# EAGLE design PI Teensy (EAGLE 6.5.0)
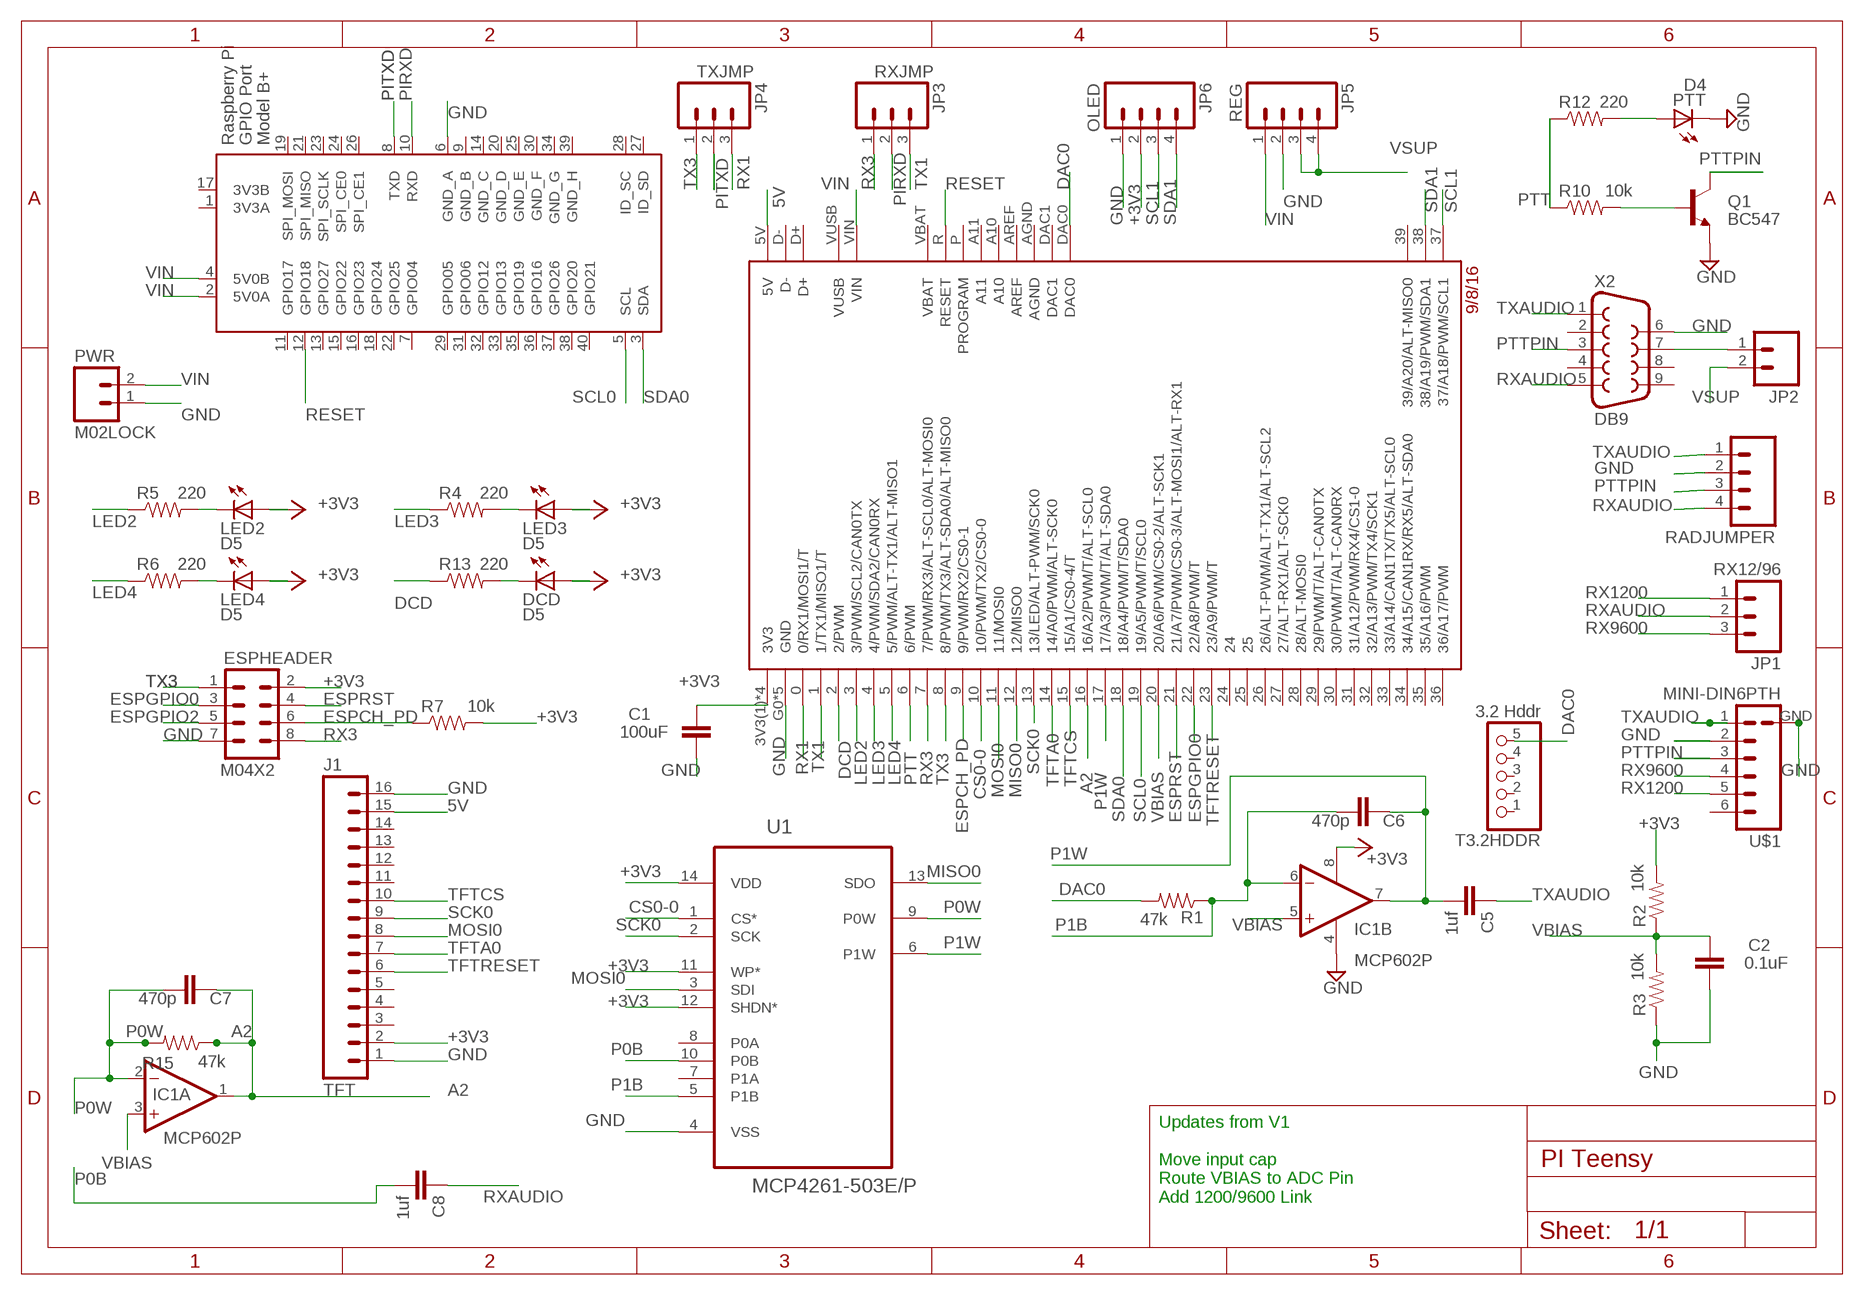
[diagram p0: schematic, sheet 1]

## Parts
C1  100uF  CAP_  [AXIAL-5MM]
C2  0.1uF  CAP_  [AXIAL-5MM]
C5  1uf  CAP_  [AXIAL-5MM]
C6  470p  CAP_  [AXIAL-5MM]
C7  470p  CAP_  [AXIAL-5MM]
C8  1uf  CAP_  [AXIAL-5MM]
DCD  D5  LED3MM  [LED3MM]
ESPHEADER  M04X2  [2X4]
IC1  MCP602P  [DIL08]
J1  TFT  M16LOCK  [1X16_LOCK]
JP1  RX12/96  M03LOCK  [1X03_LOCK]
JP2  M02LOCK  [1X02_LOCK]
JP3  RXJMP  M03LOCK  [1X03_LOCK]
JP4  TXJMP  M03LOCK  [1X03_LOCK]
JP5  REG  M04LOCK_LONGPADS  [1X04_LOCK_LONGPADS]
JP6  OLED  M04LOCK_LONGPADS  [1X04_LOCK_LONGPADS]
LED2  D5  LED3MM  [LED3MM]
LED3  D5  LED3MM  [LED3MM]
LED4  D5  LED3MM  [LED3MM]
PTT  D4  LED3MM  [LED3MM]
PWR  M02LOCK  [1X02_LOCK]
Q1  BC547  TRANSISTOR_NPNBC547  [TO-92-AMMO]
R1  47k  RESISTORAXIAL-0.3  [AXIAL-0.3]
R2  10k  RESISTOREZ  [AXIAL-0.3EZ]
R3  10k  RESISTORAXIAL-0.3  [AXIAL-0.3]
R4  220  RESISTORPTH-1/6W  [1/6W-RES]
R5  220  RESISTORPTH-1/6W  [1/6W-RES]
R6  220  RESISTORPTH-1/6W  [1/6W-RES]
R7  10k  RESISTORPTH-1/6W  [1/6W-RES]
R10  10k  RESISTORAXIAL-0.3  [AXIAL-0.3]
R12  220  RESISTORPTH-1/6W  [1/6W-RES]
R13  220  RESISTORPTH-1/6W  [1/6W-RES]
R15  47k  RESISTORAXIAL-0.3  [AXIAL-0.3]
RADJUMPER  M04LOCK  [1X04_LOCK]
T3.2HDDR  3.2 Hddr  PINHD-1X5  [1X05]
U1  MCP4261-503E/P  [DIP254P762X533-14]
U$1  MINI-DIN6PTH  [MINI-DIN6]
U$2  TEENSY3_6--ALLPINS  [T36]
X1  RASPI_BOARD_B+#_FP  [RASPI_BOARD_B+_FULL_PAD]
X2  DB9  DB9FEMALE  [DB9]

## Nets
5V [power]: J1.15 U$2.5V
+3V3 [3v3]: C1.P$1 DCD.A ESPHEADER.2 IC1.8(P:V+) J1.2 JP6.2 LED2.A LED3.A LED4.A R2.P$2 R7.2 U1.11(WP*) U1.12(SHDN*) U1.14(VDD) U$2.3V3(1)(3V3) U$2.3V3(2)(3V3) U$2.3V3(3)(3V3) U$2.3V3(4)(3V3)
A2: C7.P$1 IC1.1(A:OUT) R15.P$1 U$2.16(16/A2/PWM/T/ALT-SCL0)
CS0-0: U1.1(CS*) U$2.10(10/PWM/TX2/CS0-0)
DAC0: R1.P$2 T3.2HDDR.5 U$2.DAC0
DCD: R13.1 U$2.2(2/PWM)
ESPCH_PD: ESPHEADER.6 R7.1 U$2.9(9/PWM/RX2/CS0-1)
ESPGPIO0: ESPHEADER.3 U$2.22(22/A8/PWM/T)
ESPGPIO2: ESPHEADER.5
ESPRST: ESPHEADER.4 U$2.21(21/A7/PWM/CS0-3/ALT-MOSI1/ALT-RX1)
GND: C1.P$2 C2.P$2 ESPHEADER.7 IC1.4(P:V-) J1.1 J1.16 JP5.2 JP6.1 PTT.K(C) PWR.1 Q1.3(E) R3.P$1 RADJUMPER.2 U1.4(VSS) U$1.2 U$1.GND U$2.G0(GND) U$2.G1(GND) U$2.G2(GND) U$2.G4(GND) U$2.G5(GND) X1.6(GND_A) X2.6
LED2: R5.1 U$2.3(3/PWM/SCL2/CAN0TX)
LED3: R4.1 U$2.4(4/PWM/SDA2/CAN0RX)
LED4: R6.1 U$2.5(5/PWM/ALT-TX1/ALT-MISO1)
MISO0: U1.13(SDO) U$2.12(12/MISO0)
MOSI0: J1.8 U1.3(SDI) U$2.11(11/MOSI0)
N$1: PTT.A R12.2
N$2: Q1.2(B) R10.P$2
N$3: LED4.K(C) R6.2
N$4 [power]: JP2.1 X2.7
N$5: LED3.K(C) R4.2
N$6: LED2.K(C) R5.2
N$13: DCD.K(C) R13.2
P0B: C8.P$2 U1.10(P0B)
P0W: C7.P$2 IC1.2(A:-IN) R15.P$2 U1.9(P0W)
P1B: C6.P$2 IC1.6(B:-IN) R1.P$1 U1.5(P1B)
P1W: C5.P$2 C6.P$1 IC1.7(B:OUT) U1.6(P1W) U$2.17(17/A3/PWM/T/ALT-SDA0)
PIRXD: JP3.2 X1.10(RXD)
PITXD: JP4.2 X1.8(TXD)
PTT: R10.P$1 R12.1 U$2.6(6/PWM)
PTTPIN: Q1.1(C) RADJUMPER.3 U$1.3 X2.3
RESET: U$2.R(RESET) X1.12(GPIO18)
RX1: JP4.3 U$2.0(0/RX1/MOSI1/T)
RX3: ESPHEADER.8 JP3.1 U$2.7(7/PWM/RX3/ALT-SCL0/ALT-MOSI0)
RX1200: JP1.1 U$1.5
RX9600: JP1.3 U$1.4
RXAUDIO: C8.P$1 JP1.2 RADJUMPER.4 X2.5
SCK0: J1.9 U1.2(SCK) U$2.13(13/LED/ALT-PWM/SCK0)
SCL0: U$2.19(19/A5/PWM/T/SCL0) X1.5(SCL)
SCL1: JP6.3 U$2.37(37/A18/PWM/SCL1)
SDA0: U$2.18(18/A4/PWM/T/SDA0) X1.3(SDA)
SDA1: JP6.4 U$2.38(38/A19/PWM/SDA1)
TFTA0: J1.7 U$2.14(14/A0/PWM/ALT-SCK0)
TFTCS: J1.10 U$2.15(15/A1/CS0-4/T)
TFTRESET: J1.6 U$2.23(23/A9/PWM/T)
TX1: JP3.3 U$2.1(1/TX1/MISO1/T)
TX3: ESPHEADER.1 JP4.1 U$2.8(8/PWM/TX3/ALT-SDA0/ALT-MISO0)
TXAUDIO: C5.P$1 RADJUMPER.1 U$1.1 X2.1
VBIAS: C2.P$1 IC1.3(A:+IN) IC1.5(B:+IN) R2.P$1 R3.P$2 U$2.20(20/A6/PWM/CS0-2/ALT-SCK1)
VIN [power]: JP5.1 PWR.2 U$2.VIN X1.2(5V0A) X1.4(5V0B)
VSUP [power]: JP2.2 JP5.3 JP5.4
Unconnected: J1.3 J1.4 J1.5 J1.11 J1.12 J1.13 J1.14 T3.2HDDR.1 T3.2HDDR.2 T3.2HDDR.3 T3.2HDDR.4 U1.7(P1A) U1.8(P0A) U$1.6 U$2.24 U$2.25 U$2.26(26/ALT-PWM/ALT-TX1/ALT-SCL2) U$2.27(27/ALT-RX1/ALT-SCK0) U$2.28(28/ALT-MOSI0) U$2.29(29/PWM/T/ALT-CAN0TX) U$2.30(30/PWM/T/ALT-CAN0RX) U$2.31(31/A12/PWM/RX4/CS1-0) U$2.32(32/A13/PWM/TX4/SCK1) U$2.33(33/A14/CAN1TX/TX5/ALT-SCL0) U$2.34(34/A15/CAN1RX/RX5/ALT-SDA0) U$2.35(35/A16/PWM) U$2.36(36/A17/PWM) U$2.39(39/A20/ALT-MISO0) U$2.A10 U$2.A11 U$2.AGND U$2.AREF U$2.D+ U$2.D- U$2.DAC1 U$2.P(PROGRAM) U$2.VBAT U$2.VUSB X1.7(GPIO04) X1.11(GPIO17) X1.13(GPIO27) X1.15(GPIO22) X1.16(GPIO23) X1.18(GPIO24) X1.19(SPI_MOSI) X1.21(SPI_MISO) X1.22(GPIO25) X1.23(SPI_SCLK) X1.24(SPI_CE0) X1.26(SPI_CE1) X1.27(ID_SD) X1.28(ID_SC) X1.29(GPIO05) X1.31(GPIO06) X1.32(GPIO12) X1.33(GPIO13) X1.35(GPIO19) X1.36(GPIO16) X1.37(GPIO26) X1.38(GPIO20) X1.40(GPIO21) X2.2 X2.4 X2.8 X2.9

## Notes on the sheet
- Updates from V1
  
  Move input cap
  Route VBIAS to ADC Pin
  Add 1200/9600 Link

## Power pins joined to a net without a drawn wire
3V3A: X1.1(3V3A)
3V3B: X1.17(3V3B)
GND_B: X1.9(GND_B)
GND_C: X1.14(GND_C)
GND_D: X1.20(GND_D)
GND_E: X1.25(GND_E)
GND_F: X1.30(GND_F)
GND_G: X1.34(GND_G)
GND_H: X1.39(GND_H)

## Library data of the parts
C1 C2 C5-C8 = SparkFun-Passives:CAP: Capacitor
DCD LED2-LED4 PTT = led:LED: LED
ESPHEADER = SparkFun-Connectors:M04X2: .1" header, two rows of four.
IC1 = linear:MCP602: Single Op Amp 2.7V to 6.0V Single Supply CMOS Source: http://ww1.microchip.com/downloads/en/DeviceDoc/21314g.pdf
J1 = SparkFun-Connectors:M16: 1x16 .1" header
JP1 JP3 JP4 = SparkFun-Connectors:M03: Header 3 Standard 3-pin 0.1" header. Use with straight break away headers (SKU : PRT-00116), right angle break away headers (PRT-00553), swiss pins (PRT-00743), machine pins (PRT-00117), and female headers (PRT-00115). Molex polarized connector foot print use with SKU : PRT-08232 with associated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
JP2 PWR = SparkFun-Connectors:M02: Standard 2-pin 0.1" header. Use with
JP5 JP6 RADJUMPER = SparkFun-Connectors:M04: Header 4 Standard 4-pin 0.1" header. Use with straight break away headers (SKU : PRT-00116), right angle break away headers (PRT-00553), swiss pins (PRT-00743), machine pins (PRT-00117), and female headers (PRT-00115). Molex polarized connector foot print use with SKU : PRT-08231 with associated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
Q1 = SparkFun-DiscreteSemi:TRANSISTOR_NPN: Generic NPN BJT MMBT2222A - TRANS-08049 (SOT-23, 1A 40V) MPSA42 - TRANS-09116 (SOT-23, 500mA 300V) MMBT5088LT1G - TRANS-11160 (SOT-23, 50 mA 30V) BC547 - COM-08928 (TO-92 45V 100mA) (1.Collector 2.Base 3.Emitter) 2N3904 - COM-00521 (TO-92 40V 200mA) (1.Emitter 2.Base 3.Collector) P2N2222A -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
R1-R7 R10 R12 R13 R15 = SparkFun-Resistors:RESISTOR: Resistor
T3.2HDDR = pinhead:PINHD-1X5: PIN HEADER
U1 = MCP4261:MCP4261-503E/P: IC DGTL POT 50K 2CH ,DIP-14; MPN: MCP4261-503E/P; OC_FARNELL: 1840731; OC_NEWARK: 27M0192; PACKAGE: DIP-14; SUPPLIER: Microchip
U$1 = SparkFun-Connectors:MINI-DIN6: mini DIN 6 Connector Commonly found on the back of a computer for PS2 keyboard and mice. Schematic and footprint are proven. Spark Fun Electronics SKU : PRT-08509
U$2 = Teensy_3_6:TEENSY3_6--ALLPINS
X1 = raspberrypi_bastelstube_v13:RASPI_BOARD_B+#: Raspberry Pi GPIO connector with markings for the outer dimensions of the Raspberry Pi board model B+ with different sets of drill holes or mounting pads All pins connected
X2 = SparkFun-Connectors:DB9: DB9 Connector Standard DB9 (D-Sub 9) serial connector. Can be used for CAN bus as well as RS485 and RS232. Footprint production proven. Spark Fun Electronics SKU : PRT-00429

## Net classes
1 power: width 0.406 mm
2 3v3: width 0.305 mm

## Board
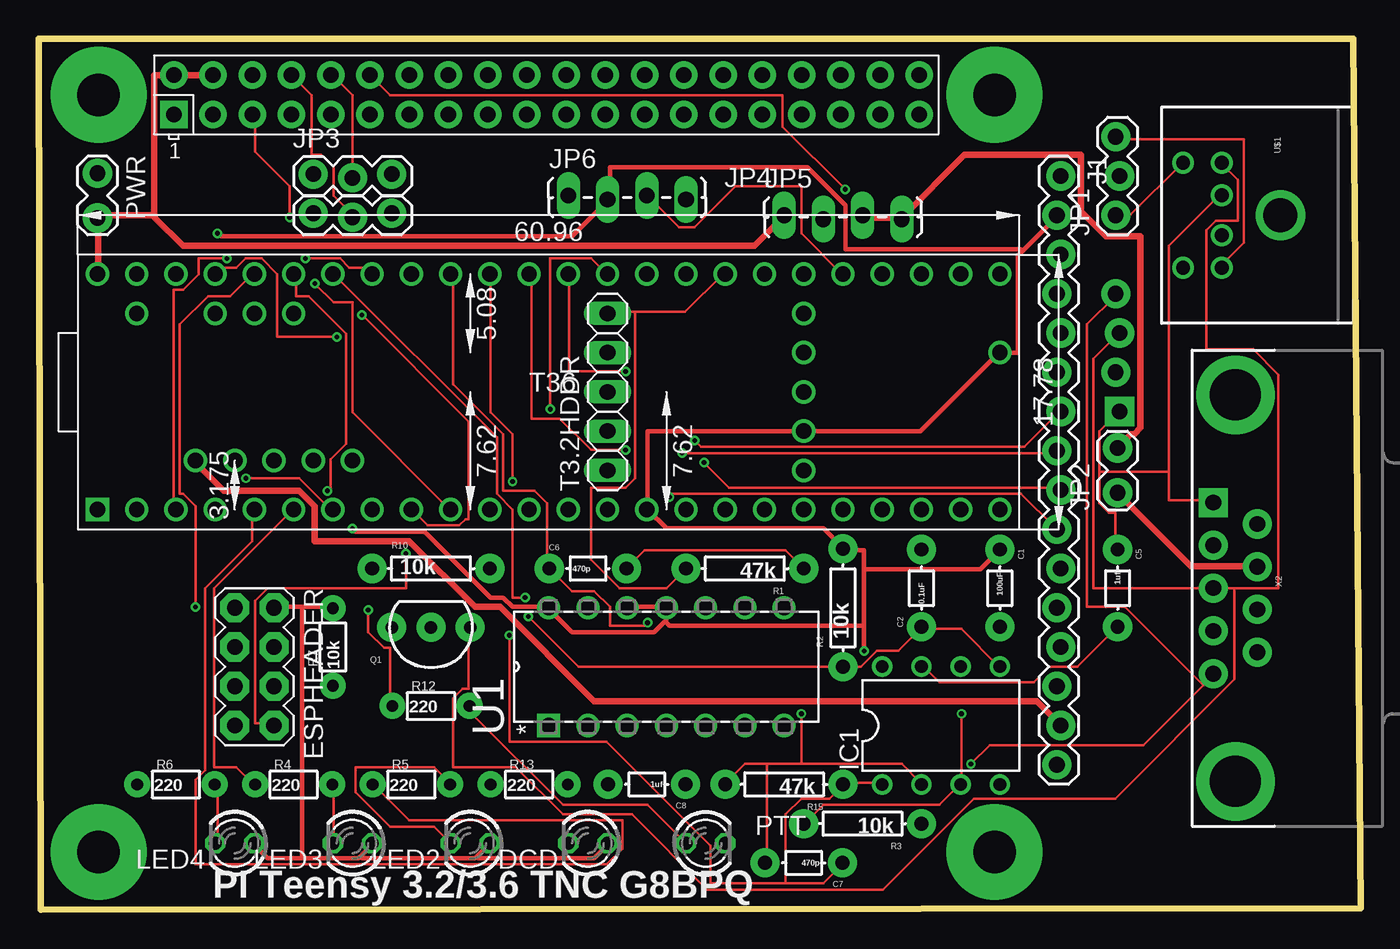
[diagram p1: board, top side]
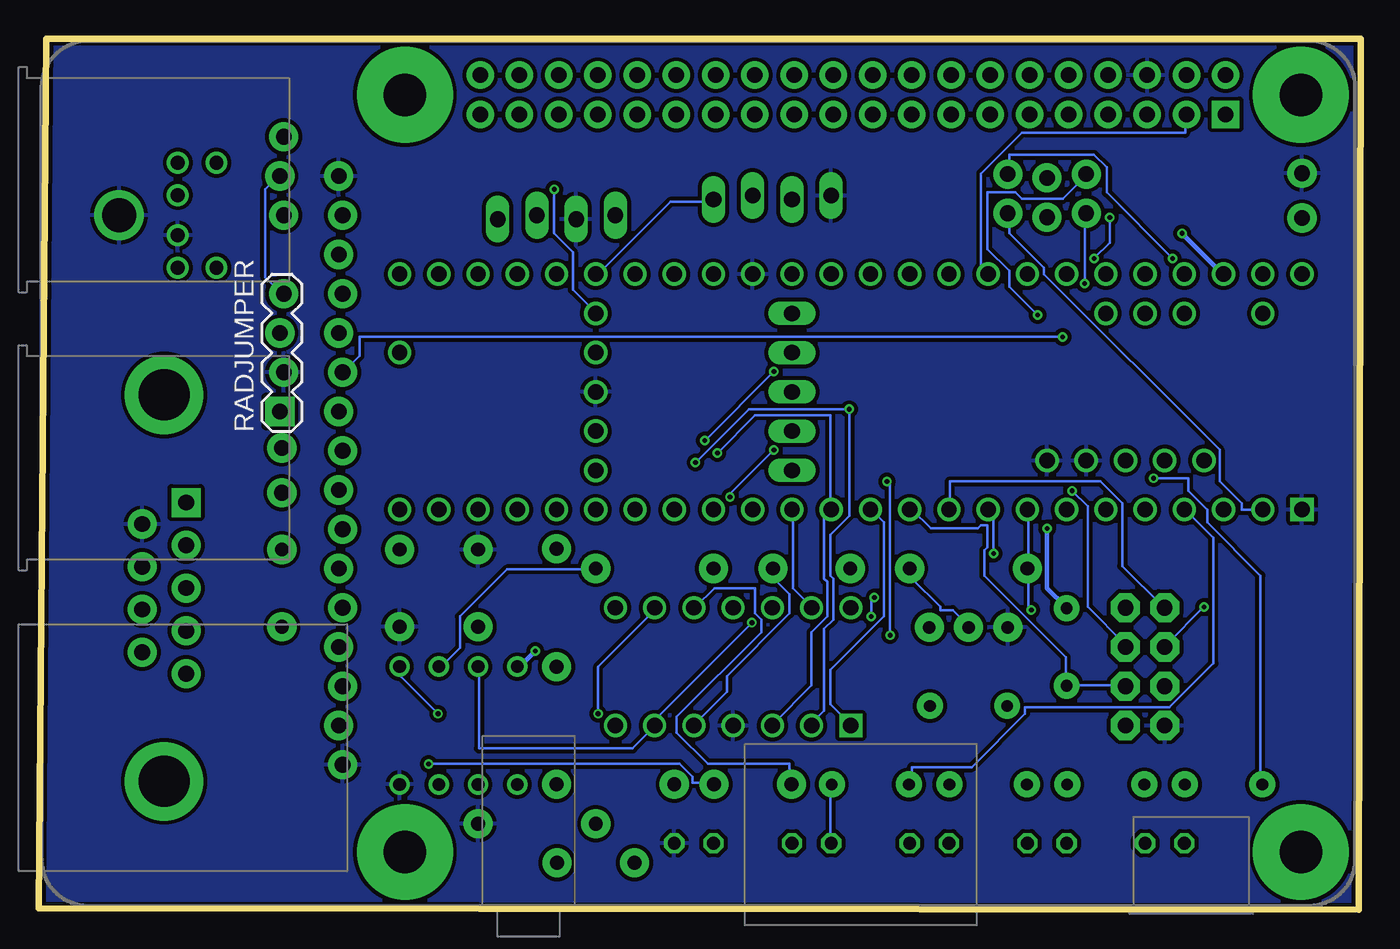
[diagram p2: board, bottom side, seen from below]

Size 85.6 x 56.39 mm. Coordinates in mm from the lower left corner, seen from the top.
Outline: 0,56.39 85.09,56.39 85.6,0.13 0.13,0 0,56.39
Copper layers (1*16): Top 0.035mm / dielectric 1.5mm / Bottom 0.035mm
Design rules "SeeedStudio_2layer_DRU_no_angle_20140221": minimum track width 6mil, minimum drill 12mil, track to track 6mil, track to pad 6mil, pad to pad 6mil, via to via 6mil, smd to smd 0mil, copper to edge 10mil, drill to drill 10mil, minimum pad ring 10mil, minimum via ring 6mil, stop-mask expansion 2mil, vias tented up to drill 100mil, thermal gap 10mil

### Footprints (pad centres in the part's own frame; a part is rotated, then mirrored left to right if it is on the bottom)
AXIAL-5MM = drill 0.9 pad 1.88: P$1 -2.5,0; P$2 2.5,0
LED3MM = drill 0.813 octagon: A -1.27,0; K 1.27,0
2X4 = drill 1.016 pad 1.88 octagon: 1 -3.81,-1.27; 2 -3.81,1.27; 3 -1.27,-1.27; 4 -1.27,1.27; 5 1.27,-1.27; 6 1.27,1.27; 7 3.81,-1.27; 8 3.81,1.27
DIL08 = drill 0.813 pad 1.27: 1 -3.81,-3.81; 2 -1.27,-3.81; 3 1.27,-3.81; 4 3.81,-3.81; 5 3.81,3.81; 6 1.27,3.81; 7 -1.27,3.81; 8 -3.81,3.81
1X16_LOCK = drill 1.016 pad 1.88: 1 0,0.127; 2 2.54,-0.127; 3 5.08,0.127; 4 7.62,-0.127; 5 10.16,0.127; 6 12.7,-0.127; 7 15.24,0.127; 8 17.78,-0.127; 9 20.32,0.127; 10 22.86,-0.127; 11 25.4,0.127; 12 27.94,-0.127; 13 30.48,0.127; 14 33.02,-0.127; 15 35.56,0.127; 16 38.1,-0.127
1X03_LOCK = drill 1.016 pad 1.88: 1 0,0.127; 2 2.54,-0.127; 3 5.08,0.127
1X02_LOCK = drill 1.016 pad 1.88: 1 -0.178,0; 2 2.718,0
1X04_LOCK_LONGPADS = drill 1.016 long: 1 0,0; 2 2.54,-0.254; 3 5.08,0; 4 7.62,-0.254
TO-92-AMMO = drill 0.813 pad 1.88: 1 -2.54,0; 2 0,0; 3 2.54,0
AXIAL-0.3 = drill 0.9 pad 1.88: P$1 -3.81,0; P$2 3.81,0
AXIAL-0.3EZ = drill 0.9 pad 1.88: P$1 -3.81,0; P$2 3.81,0
1/6W-RES = drill 0.762 pad 1.676: 1 -2.5,0; 2 2.5,0
1X04_LOCK = drill 1.016 pad 1.88 square: 1 0,0.127 | drill 1.016 pad 1.88: 2 2.54,-0.127; 3 5.08,0.127; 4 7.62,-0.127
1X05 = drill 1.016 long: 1 -5.08,0; 2 -2.54,0; 3 0,0; 4 2.54,0; 5 5.08,0
DIP254P762X533-14 = drill 0.991 square: 1 -7.62,15.24 | drill 0.991: 2 -7.62,12.7; 3 -7.62,10.16; 4 -7.62,7.62; 5 -7.62,5.08; 6 -7.62,2.54; 7 -7.62,0; 8 0,0; 9 0,2.54; 10 0,5.08; 11 0,7.62; 12 0,10.16; 13 0,12.7; 14 0,15.24
MINI-DIN6 = drill 0.9: 1 -1.3,-8.5; 2 1.3,-8.5; 3 -3.4,-8.5; 4 3.4,-8.5; 5 -3.4,-11; 6 3.4,-11 | drill 2.2: GND 0,-4.7
T36 = drill 1: 0 -15.24,-5.08; 1 -12.7,-5.08; 2 -10.16,-5.08; 3 -7.62,-5.08; 3V3(1) 17.78,-5.08; 3V3(2) 27.94,0; 3V3(3) -12.7,10.16; 3V3(4) 40.64,5.08; 4 -5.08,-5.08; 5 -2.54,-5.08; 5V -11.43,-1.905; 6 0,-5.08; 7 2.54,-5.08; 8 5.08,-5.08; 9 7.62,-5.08; 10 10.16,-5.08; 11 12.7,-5.08; 12 15.24,-5.08; 13 15.24,10.16; 14 12.7,10.16; 15 10.16,10.16; 16 7.62,10.16; 17 5.08,10.16; 18 2.54,10.16; 19 0,10.16; 20 -2.54,10.16; 21 -5.08,10.16; 22 -7.62,10.16; 23 -10.16,10.16; 24 20.32,-5.08; 25 22.86,-5.08; 26 25.4,-5.08; 27 27.94,-5.08; 28 30.48,-5.08; 29 33.02,-5.08; 30 35.56,-5.08; 31 38.1,-5.08; 32 40.64,-5.08; 33 40.64,10.16; 34 38.1,10.16; 35 35.56,10.16; 36 33.02,10.16; 37 30.48,10.16; 38 27.94,10.16; 39 25.4,10.16; A10 -7.62,7.62; A11 -5.08,7.62; AGND -15.24,10.16; AREF -10.16,7.62; D+ -6.35,-1.905; D- -8.89,-1.905; DAC0 22.86,10.16; DAC1 20.32,10.16; G1 27.94,2.54; G2 17.78,10.16; G4 -3.81,-1.905; G5 -1.27,-1.905; P 27.94,5.08; R 27.94,7.62; VBAT 27.94,-2.54; VIN -17.78,10.16; VUSB -15.24,7.62 | drill 1 square: G0 -17.78,-5.08
RASPI_BOARD_B+_FULL_PAD = drill 1 pad 1.778 square: 1 8.37,51.23 | drill 1 pad 1.778: 2 8.37,53.77; 3 10.91,51.23; 4 10.91,53.77; 5 13.45,51.23; 6 13.45,53.77; 7 15.99,51.23; 8 15.99,53.77; 9 18.53,51.23; 10 18.53,53.77; 11 21.07,51.23; 12 21.07,53.77; 13 23.61,51.23; 14 23.61,53.77; 15 26.15,51.23; 16 26.15,53.77; 17 28.69,51.23; 18 28.69,53.77; 19 31.23,51.23; 20 31.23,53.77; 21 33.77,51.23; 22 33.77,53.77; 23 36.31,51.23; 24 36.31,53.77; 25 38.85,51.23; 26 38.85,53.77; 27 41.39,51.23; 28 41.39,53.77; 29 43.93,51.23; 30 43.93,53.77; 31 46.47,51.23; 32 46.47,53.77; 33 49.01,51.23; 34 49.01,53.77; 35 51.55,51.23; 36 51.55,53.77; 37 54.09,51.23; 38 54.09,53.77; 39 56.63,51.23; 40 56.63,53.77 | drill 2.75 pad 6.2: DRILL_1 3.5,52.5; DRILL_2 61.5,52.5; DRILL_3 3.5,3.5; DRILL_4 61.5,3.5
DB9 = drill 1.016 pad 1.88 square: 1 -5.54,-1.42 | drill 1.016 pad 1.88: 2 -2.77,-1.42; 3 0,-1.42; 4 2.77,-1.42; 5 5.54,-1.42; 6 -4.15,1.42; 7 -1.38,1.42; 8 1.38,1.42; 9 4.15,1.42 | drill 3.302 pad 5.08: G1 -12.5,0; G2 12.5,0

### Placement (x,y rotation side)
C1  62.23,20.83 270 top
C2  57.15,20.83 90 top
C5  69.85,20.83 270 top
C6  35.56,22.1 0 top
C7  49.53,3.05 180 top
C8  39.37,8.13 180 top
DCD  35.56,4.32 180 top
ESPHEADER  13.97,15.75 270 top
IC1  58.42,11.94 0 top
J1  66.04,47.5 270 top
JP1  69.85,44.96 90 top
JP2  69.85,27.18 90 top
JP3  17.78,47.5 0 top
JP4  17.78,44.96 0 top
JP5  48.26,44.96 0 top
JP6  34.29,46.23 0 top
LED2  27.94,4.32 180 top
LED3  20.32,4.32 180 top
LED4  12.7,4.32 180 top
PTT  43.18,4.32 0 top
PWR  3.81,47.5 270 top
Q1  25.4,18.29 180 top
R1  45.72,22.1 180 top
R2  52.07,19.56 90 top
R3  53.34,5.59 180 top
R4  16.51,8.13 0 top
R5  24.13,8.13 0 top
R6  8.89,8.13 0 top
R7  19.05,17.02 90 top
R10  25.4,22.1 0 top
R12  25.4,13.21 0 top
R13  31.75,8.13 0 top
R15  48.26,8.13 180 top
RADJUMPER  69.85,32.26 90 bottom
T3.2HDDR  36.83,33.53 90 top
U1  48.26,19.56 90 top
U$1  85.09,44.96 270 top
U$2  21.59,30.99 0 top
X1  0.38,0.25 0 top
X2  77.47,20.83 270 top

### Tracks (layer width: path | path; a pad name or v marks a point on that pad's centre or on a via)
5V
  Top 0.406: U$2.5V 10.16,28.96 11.99,27.13 16.87,27.13 17.88,26.11 17.88,23.88 23.98,23.88 28.25,19.61 29.87,19.61 35.97,13.51 64.62,13.51 66.04,12.09 J1.15
+3V3  (via drill 0.3)
  Top 0.305: 17.07,19.61 15.24,19.61 ESPHEADER.2 | 17.07,19.61 18.9,19.61 R7.2 | 17.07,3.35 20.73,3.35 20.83,3.45 | 17.07,3.35 14.83,3.35 14.02,4.17 LED4.A | 20.83,3.45 21.54,4.17 LED3.A | 28.35,3.45 28.25,3.35 20.93,3.35 20.83,3.45 | 28.35,3.45 LED2.A | DCD.A 36.78,4.17 35.97,3.35 28.45,3.35 28.35,3.45 | 17.07,3.35 17.07,19.61 | 40.54,18.69 40.64,18.8 U1.11 40.64,19.61 38.2,19.61 U1.12 | 40.54,18.69 39.83,17.98 34.54,17.98 33.12,19.41 U1.14 32.92,19.61 30.68,19.61 30.07,20.22 29.26,20.22 24.99,24.49 20.52,24.49 v20.32,24.69 | 53.44,22.05 53.44,23.27 52.22,23.27 R2.P$2 52.02,23.47 50.8,24.69 40.64,24.69 39.42,25.91 | 53.44,22.05 53.44,18.39 | 53.44,18.39 v53.44,16.76 | 53.44,22.05 60.96,22.05 62.18,23.27 C1.P$1 | 40.54,18.69 40.84,18.39 53.44,18.39 | v11.58,43.79 11.79,43.59 34.54,43.59 36.78,45.82 JP6.2 36.98,46.03 36.98,48.06 49.78,48.06 52.22,45.62 52.22,42.77 63.6,42.77 63.7,42.67 | 39.42,25.91 39.42,30.99 U$2.3V3(2) 57.1,30.99 62.18,36.07 U$2.3V3(4) 63.4,36.07 63.4,42.37 63.7,42.67 | 63.7,42.67 65.84,44.81 J1.2 | 39.42,25.91 U$2.3V3(1)
  Bottom 0.305: v53.44,16.76 54.46,15.75 IC1.8 | v11.58,43.79 8.94,41.15 U$2.3V3(3) | v20.32,24.69 20.32,20.83 19.1,19.61 R7.2
A2  (via drill 0.3)
  Top 0.152: IC1.1 54.46,8.23 52.22,8.23 R15.P$1 52.02,8.03 51.21,7.21 49.38,7.21 48.36,6.2 48.36,1.73 | v30.68,27.74 30.68,30.79 29.26,32.21 29.26,41.15 U$2.16 | v30.48,17.78 30.48,10.87 36.78,10.87 43.48,4.17 43.48,1.73 48.36,1.73 | 48.36,1.73 50.8,1.73 52.02,2.95 C7.P$1
  Bottom 0.152: v30.68,27.74 30.48,27.53 v30.48,17.78
CS0-0
  Bottom 0.152: U1.1 33.12,12.09 34.34,13.31 34.34,15.55 30.89,19 30.89,25.09 31.7,25.91 U$2.10
DAC0
  Top 0.152: 38.61,38.71 36.98,38.71 T3.2HDDR.5 | 38.61,38.71 41.86,38.71 44.3,41.15 U$2.DAC0 | R1.P$2 40.64,20.83 37.59,20.83 35.76,22.66 35.76,27.33 38,27.33 38.61,27.94 38.61,38.71
DCD
  Bottom 0.152: U$2.2 11.38,25.91 9.55,24.08 9.55,15.95 12.39,13.11 21.74,13.11 21.74,12.7 25.2,9.25 29.06,9.25 29.06,8.23 R13.1
ESPCH_PD
  Bottom 0.152: U$2.9 29.06,25.91 27.84,24.69 24.79,24.69 24.59,24.89 24.18,24.89 24.18,23.47 24.38,23.27 24.38,21.64 19.1,16.36 19.1,14.53 R7.1 18.9,14.53 15.24,14.53 ESPHEADER.6
ESPGPIO0  (via drill 0.3)
  Top 0.152: v10.16,19.61 10.16,26.11 9.35,26.92 9.14,26.92 9.14,37.9 10.97,39.73 12.39,39.73 13.82,41.15 U$2.22
  Bottom 0.152: v10.16,19.61 12.6,17.17 ESPHEADER.3
ESPRST  (via drill 0.3)
  Top 0.152: v18.69,27.13 18.9,27.13 18.9,29.16 19.91,30.18 19.91,37.29 17.48,39.73 16.66,39.73 16.66,41.15 U$2.21
  Bottom 0.152: v18.69,27.13 17.68,26.11 17.68,19.61 15.24,17.17 ESPHEADER.4
GND
  pour Bottom (isolate 0.254): 0.25,0.13 0,56.39 85.09,56.39 85.6,0.13
LED2
  Top 0.152: U$2.3 13.82,25.91 13.82,23.88 10.77,20.83 10.77,9.04 10.16,8.43 10.16,2.95 36.78,2.95 37.8,3.96 37.8,5.79 23.98,5.79 21.74,8.03 R5.1
LED3
  Top 0.152: U$2.4 16.46,25.91 11.38,20.83 11.38,9.25 12.8,9.25 13.82,8.23 R4.1
LED4  (via drill 0.3)
  Top 0.152: v13.41,27.94 16.87,27.94 18.9,25.91 U$2.5
  Bottom 0.152: v13.41,27.94 11.18,27.94 11.18,27.13 9.96,25.91 9.96,25.09 6.5,21.64 6.5,8.23 R6.1
MISO0
  Bottom 0.152: U1.13 35.56,19.61 36.78,20.83 36.78,25.91 U$2.12
MOSI0  (via drill 0.3)
  Top 0.152: v41.66,29.57 65.84,29.57 J1.8
  Bottom 0.152: 34.34,25.91 34.75,25.5 34.75,21.44 34.54,21.23 34.54,19 35.56,17.98 35.56,14.53 38,12.09 U1.3 | v41.66,29.57 39.22,32 34.34,32 34.34,25.91 | 34.34,25.91 U$2.11
N$1
  Top 0.152: PTT.A 39.42,6.81 33.93,6.81 28.04,12.7 28.04,13.11 R12.2
N$2
  Bottom 0.152: Q1.2 25.4,18.39 26.42,19.41 27.23,19.41 27.23,19.61 29.06,21.44 29.06,22.05 R10.P$2
N$3
  Top 0.152: LED4.K 11.58,4.37 11.58,8.03 R6.2
N$4
  Top 0.406: JP2.1 69.9,26.92 74.57,22.25 78.84,22.25 X2.7
N$5
  Top 0.152: LED3.K 19.1,4.37 19.1,8.03 R4.2
N$6
  Top 0.152: LED2.K 25.6,5.38 22.76,5.38 20.52,7.62 20.52,9.25 25.6,9.25 26.62,8.23 R5.2
N$13
  Bottom 0.152: DCD.K 34.34,4.37 34.34,8.03 R13.2
P0B
  Bottom 0.152: U1.10 43.08,19.61 41.86,20.83 39.22,20.83 39.22,19.2 38.81,18.8 38.81,17.98 44.3,12.5 44.3,11.48 42.27,9.45 36.98,9.45 36.98,8.23 C8.P$2
P0W  (via drill 0.3)
  Top 0.152: 47.14,9.45 45.72,9.45 44.5,8.23 R15.P$2 | 47.14,9.45 49.38,9.45 | 49.38,9.45 55.88,9.45 57.1,8.23 IC1.2 | 49.38,9.45 v49.38,12.7 | 47.14,9.45 47.14,3.15 C7.P$2
  Bottom 0.152: v49.38,12.7 49.38,15.75 45.72,19.41 U1.9
P1B
  Top 0.152: R1.P$1 48.36,23.27 39.22,23.27 38.2,22.25 C6.P$2
  Bottom 0.152: U1.5 43.08,12.09 41.05,14.12 41.05,15.14 36.98,19.2 36.98,20.42 38,21.44 38,22.05 C6.P$2 | IC1.6 59.54,15.75 58.32,16.97 58.32,19 55.27,22.05 49.58,22.05 R1.P$1
P1W  (via drill 0.3)
  Top 0.152: U$2.17 26.82,41.15 26.82,34.04 30.07,30.79 30.07,27.13 32.11,27.13 32.92,26.31 32.92,22.25 C6.P$1 33.12,22.05 34.54,20.62 35.97,20.62 36.98,19.61 36.98,18.39 39.22,18.39 v39.42,18.59 | IC1.7 57.3,15.75 58.32,14.73 64.41,14.73 65.43,15.75 67.26,15.75 69.7,18.19 C5.P$2
  Bottom 0.152: IC1.7 57.1,15.75 57.1,10.46 47.14,10.46 45.72,11.89 U1.6 45.72,12.29 v39.42,18.59
PIRXD
  Top 0.152: JP3.2 20.32,52.73 19.1,53.95 X1.10
PITXD
  Top 0.152: X1.8 16.46,53.95 17.68,52.73 17.68,48.87 18.29,48.87 19.1,48.06 19.1,46.23 20.32,45.01 JP4.2
PTT  (via drill 0.3)
  Top 0.152: v21.34,19.41 21.34,17.98 22.35,16.97 22.76,16.97 22.76,13.31 R12.1
  Bottom 0.152: U$2.6 21.54,25.91 21.54,22.25 R10.P$1 21.54,22.05 21.54,19.61 v21.34,19.41
PTTPIN
  Top 0.152: 77.42,20.83 X2.3 68.28,20.83 68.28,35.66 69.9,37.29 RADJUMPER.3 | 77.42,20.83 80.26,20.83 80.26,34.65 78.64,36.27 75.59,36.27 75.59,43.99 76.2,44.6 77.62,44.6 77.62,47.24 76.61,48.26 U$1.3 | 77.42,20.83 77.42,14.93 69.7,7.21 60.55,7.21 54.66,1.32 43.28,1.32 38.41,6.2 33.93,6.2 30.89,9.25 26.82,9.25 26.82,13.72 27.43,14.33 27.84,14.33 27.84,18.19 Q1.1
RESET  (via drill 0.3)
  Top 0.152: v52.22,46.63 48.16,50.7 48.16,52.73 22.76,52.73 21.54,53.95 X1.12
  Bottom 0.152: v52.22,46.63 52.22,43.79 51,42.57 51,40.13 49.58,38.71 U$2.R
RX1
  Bottom 0.152: U$2.0 7.72,25.91 7.72,26.31 9.14,27.74 9.14,29.77 20.52,41.15 20.52,41.55 22.76,43.79 22.76,45.01 JP4.3
RX3  (via drill 0.3)
  Top 0.152: v23.77,23.06 23.77,20.83 14.83,20.83 14.02,20.02 14.02,12.09 15.24,12.09 ESPHEADER.8 | v20.93,38.51 27.84,31.6 27.84,25.3 27.64,25.3 27.23,24.89 25.2,24.89 24.18,25.91 U$2.7
  Bottom 0.152: v23.77,23.06 23.77,25.7 23.98,25.91 U$2.7 | v20.93,38.51 22.76,40.34 22.76,41.35 24.18,42.77 24.18,46.43 22.35,46.43 21.95,46.03 19.3,46.03 17.88,47.45 JP3.1
RX1200
  Top 0.152: U$1.5 73.97,48.26 70.71,45.01 69.9,45.01 JP1.1
RX9600
  Top 0.152: U$1.4 76.61,41.76 78.03,43.18 78.03,49.89 69.9,49.89 JP1.3
RXAUDIO  (via drill 0.3)
  Top 0.152: v60.35,9.45 61.57,10.67 71.53,10.67 75.39,14.53 | 75.39,14.53 76,15.14 X2.5 | 75.39,14.53 70.31,19.61 67.87,19.61 67.87,37.9 69.7,39.73 RADJUMPER.4
  Bottom 0.152: v60.35,9.45 44.09,9.45 43.28,8.64 43.28,8.23 42.06,8.23 C8.P$1 | JP1.2 70.1,47.45 70.92,46.63 70.92,40.95 69.9,39.93 RADJUMPER.4
SCK0  (via drill 0.3)
  Top 0.152: v33.12,32.41 33.12,42.16 35.76,42.16 36.78,41.15 U$2.13 | v43.08,28.96 44.7,27.33 66.04,27.33 J1.9
  Bottom 0.152: U1.2 35.56,12.09 34.75,12.9 34.75,18.19 34.14,18.8 34.14,21.44 34.34,21.64 34.34,24.28 33.12,25.5 v33.12,32.41 39.62,32.41 v43.08,28.96
SCL0  (via drill 0.3)
  Top 0.152: v17.27,42.16 19.51,42.16 20.12,41.55 21.13,41.55 21.54,41.15 U$2.19 | v16.26,44.81 16.26,46.84 14.02,49.07 14.02,51.31 X1.5
  Bottom 0.152: v17.27,42.16 16.26,43.18 v16.26,44.81
SCL1
  Top 0.152: U$2.37 52.02,41.15 49.38,43.79 49.38,46.84 45.11,46.84 42.47,44.2 41.45,44.2 39.42,46.23 JP6.3
SDA0
  Bottom 0.152: U$2.18 24.18,41.15 24.59,41.55 24.59,47.65 21.95,50.29 11.38,50.29 11.38,51.31 X1.3
SDA1
  Bottom 0.152: U$2.38 49.38,41.15 44.7,45.82 42.06,45.82 JP6.4
TFTA0  (via drill 0.3)
  Top 0.152: v38,34.85 34.34,34.85 34.34,41.15 U$2.14 | v42.47,30.38 42.88,29.97 63.8,29.97 66.04,32.21 J1.7
  Bottom 0.152: v42.47,30.38 v38,34.85
TFTCS  (via drill 0.3)
  Top 0.152: v38,29.77 35.76,29.77 33.73,31.8 31.9,31.8 31.9,41.15 U$2.15 | v40.84,26.72 41.05,26.92 63.6,26.92 65.84,24.69 J1.10
  Bottom 0.152: v38,29.77 40.84,26.92 v40.84,26.72
TFTRESET  (via drill 0.3)
  Top 0.152: v19.3,37.08 15.44,37.08 15.44,41.15 14.43,42.16 13.41,42.16 12.8,41.55 11.99,41.55 11.58,41.15 U$2.23
  Bottom 0.152: v19.3,37.08 64.82,37.08 64.82,35.87 65.84,34.85 J1.6
TX1  (via drill 0.3)
  Top 0.152: v12.19,42.16 10.36,42.16 10.36,41.15 9.35,40.13 8.74,40.13 8.74,25.91 U$2.1
  Bottom 0.152: v12.19,42.16 16.46,46.43 16.46,48.06 17.27,48.87 22.76,48.87 22.76,47.65 JP3.3
TX3  (via drill 0.3)
  Top 0.152: v17.88,40.54 19.1,39.32 20.32,39.32 20.32,32.21 26.62,25.91 U$2.8
  Bottom 0.152: v17.88,40.54 17.88,45.01 JP4.1 | ESPHEADER.1 12.8,19.61 15.44,22.25 15.44,26.31 16.87,27.74 26.62,27.74 26.62,25.91 U$2.8
TXAUDIO
  Top 0.152: 73.15,28.35 73.15,26.52 76,26.52 X2.1 | 73.15,28.35 73.15,42.98 76.4,46.23 U$1.1 | 68.68,28.35 68.68,26.31 69.29,25.7 69.7,25.7 69.7,23.47 C5.P$1 | 73.15,28.35 68.68,28.35 | 68.68,28.35 68.68,30.99 69.9,32.21 RADJUMPER.1
VBIAS  (via drill 0.3)
  Top 0.152: R3.P$2 49.58,5.59 50.8,6.81 58.32,6.81 59.54,8.03 IC1.3 59.74,8.23 v59.74,12.7 | IC1.5 62.18,15.75 59.74,18.19 57.3,18.19 C2.P$1 57.1,18.19 55.68,16.76 54.25,16.76 53.24,15.75 R2.P$1 34.95,15.75 v31.7,19 | v31.5,20.22 30.68,20.22 30.68,25.91 29.67,26.92 29.67,30.58 19.1,41.15 U$2.20
  Bottom 0.152: v31.5,20.22 31.7,20.02 v31.7,19 | v59.74,12.7 62.18,15.14 62.18,15.75 IC1.5
VIN
  Top 0.406: X1.4 X1.2 7.49,54.02 7.49,44.96 | 7.49,44.96 3.81,44.96 PWR.2 3.86,44.6 3.86,41.15 U$2.VIN | JP5.1 48.16,44.81 46.33,42.98 9.35,42.98 7.52,44.81 7.49,44.96
VSUP
  Top 0.406: 55.88,44.81 53.44,44.81 JP5.3 | 55.88,44.81 59.94,48.87 67.46,48.87 67.46,45.21 69.09,43.59 71.32,43.59 71.32,31.19 70.92,30.79 70.71,30.79 69.9,29.97 JP2.2 | 55.88,44.81 JP5.4

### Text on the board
tPlace: PI Teensy 3.2/3.6 TNC G8BPQ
